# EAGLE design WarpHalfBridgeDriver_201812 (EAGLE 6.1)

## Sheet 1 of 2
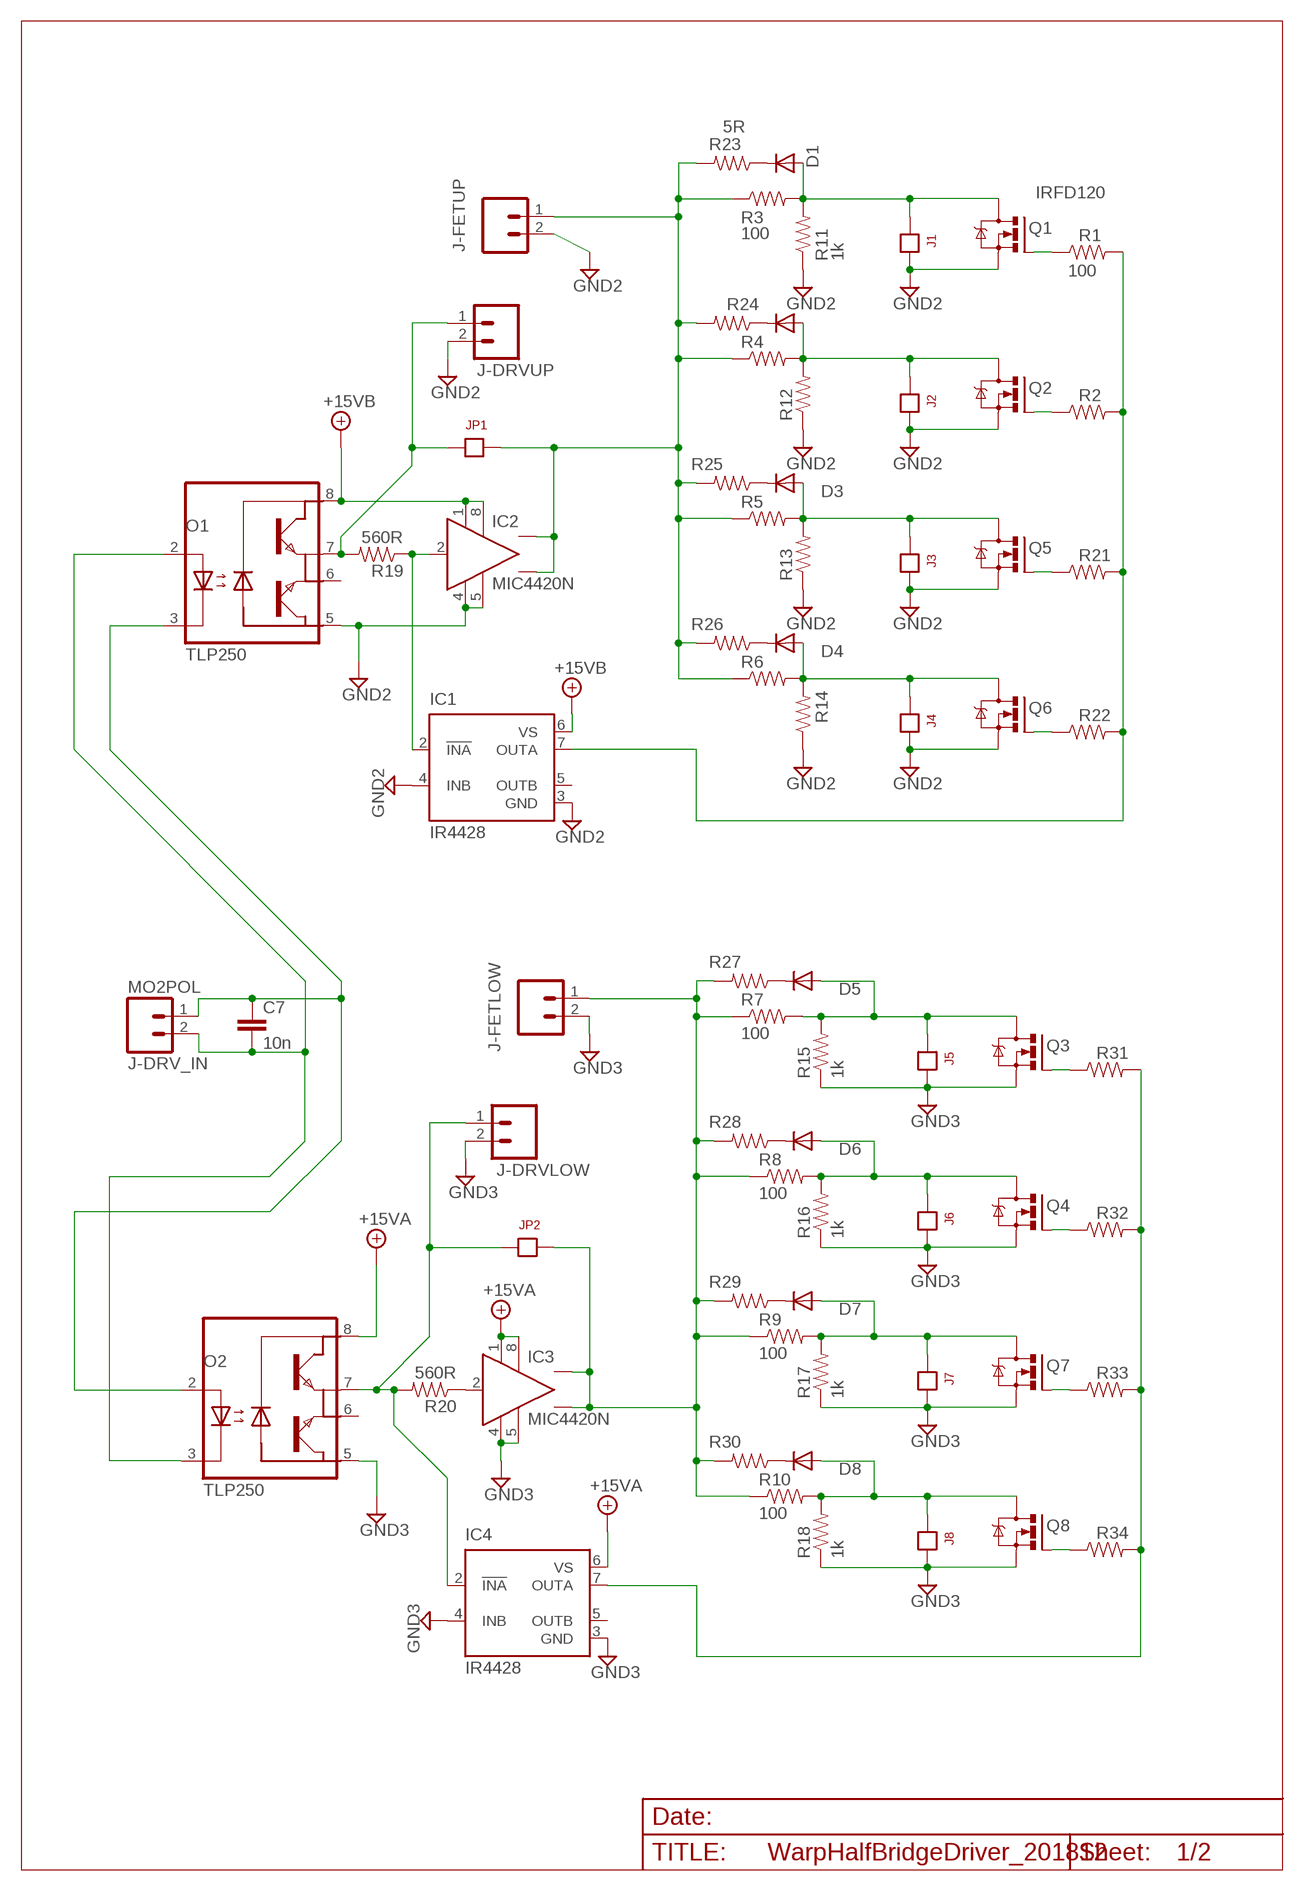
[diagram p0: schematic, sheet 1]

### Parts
C7  10n  BCAP  [BCAP]
D1  1N4004  [DO41-10]
D2  1N4004  [DO41-10]
D3  1N4004  [DO41-10]
D4  1N4004  [DO41-10]
D5  1N4004  [DO41-10]
D6  1N4004  [DO41-10]
D7  1N4004  [DO41-10]
D8  1N4004  [DO41-10]
IC1  IR4428  [DIL08]
IC2  MIC4420N  [DIL08]
IC3  MIC4420N  [DIL08]
IC4  IR4428  [DIL08]
J1  JP1  [JP1]
J2  JP1  [JP1]
J3  JP1  [JP1]
J4  JP1  [JP1]
J5  JP1  [JP1]
J6  JP1  [JP1]
J7  JP1  [JP1]
J8  JP1  [JP1]
J-DRV_IN  MO2POL  [MOLEX-1X2]
J-DRVLOW  MO2POL  [MOLEX-1X2]
J-DRVUP  MO2POL  [MOLEX-1X2]
J-FETLOW  MO2POL  [MOLEX-1X2]
J-FETUP  MO2POL  [MOLEX-1X2]
JP1  JP1  [JP1]
JP2  JP1  [JP1]
O1  TLP250  TLP250DIP8-L39  [DIL08-L39]
O2  TLP250  TLP250DIP8-L39  [DIL08-L39]
Q1  IRFD120  [DIL04]
Q2  IRFD120  [DIL04]
Q3  IRFD120  [DIL04]
Q4  IRFD120  [DIL04]
Q5  IRFD120  [DIL04]
Q6  IRFD120  [DIL04]
Q7  IRFD120  [DIL04]
Q8  IRFD120  [DIL04]
R1  100  RESISTORPTH-1/4W  [AXIAL-0.4]
R2  100  RESISTORPTH-1/4W  [AXIAL-0.4]
R3  100  RESISTORPTH-1/4W  [AXIAL-0.4]
R4  100  RESISTORPTH-1/4W  [AXIAL-0.4]
R5  100  RESISTORPTH-1/4W  [AXIAL-0.4]
R6  100  RESISTORPTH-1/4W  [AXIAL-0.4]
R7  100  RESISTORPTH-1/4W  [AXIAL-0.4]
R8  100  RESISTORPTH-1/4W  [AXIAL-0.4]
R9  100  RESISTORPTH-1/4W  [AXIAL-0.4]
R10  100  RESISTORPTH-1/4W  [AXIAL-0.4]
R11  1k  R4  [AXIAL-0.4]
R12  1k  R4  [AXIAL-0.4]
R13  1k  R4  [AXIAL-0.4]
R14  1k  R4  [AXIAL-0.4]
R15  1k  R4  [AXIAL-0.4]
R16  1k  R4  [AXIAL-0.4]
R17  1k  R4  [AXIAL-0.4]
R18  1k  R4  [AXIAL-0.4]
R19  560R  R4  [AXIAL-0.4]
R20  560R  R4  [AXIAL-0.4]
R21  100  RESISTORPTH-1/4W  [AXIAL-0.4]
R22  100  RESISTORPTH-1/4W  [AXIAL-0.4]
R23  5R  R4  [AXIAL-0.4]
R24  5R  R4  [AXIAL-0.4]
R25  5R  R4  [AXIAL-0.4]
R26  5R  R4  [AXIAL-0.4]
R27  5R  R4  [AXIAL-0.4]
R28  5R  R4  [AXIAL-0.4]
R29  5R  R4  [AXIAL-0.4]
R30  5R  R4  [AXIAL-0.4]
R31  100  RESISTORPTH-1/4W  [AXIAL-0.4]
R32  100  RESISTORPTH-1/4W  [AXIAL-0.4]
R33  100  RESISTORPTH-1/4W  [AXIAL-0.4]
R34  100  RESISTORPTH-1/4W  [AXIAL-0.4]

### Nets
+15VA: IC3.1(VS) IC3.8(VS1) IC4.6(VS) O2.8(VCC) ; also sheet 2
+15VB: IC1.6(VS) IC2.1(VS) IC2.8(VS1) O1.8(VCC) ; also sheet 2
GND2: IC1.3(GND) IC1.4(INB) IC2.4(GND) IC2.5(GND1) J1.2 J2.2 J3.2 J4.2 J-DRVUP.2 J-FETUP.2 O1.5(GND) Q1.4(S) Q2.4(S) Q5.4(S) Q6.4(S) R11.P$1 R12.P$1 R13.P$1 R14.P$1 ; also sheet 2
GND3: IC3.4(GND) IC3.5(GND1) IC4.3(GND) IC4.4(INB) J5.2 J6.2 J7.2 J8.2 J-DRVLOW.2 J-FETLOW.2 O2.5(GND) Q3.4(S) Q4.4(S) Q7.4(S) Q8.4(S) R15.P$1 R16.P$1 R17.P$1 R18.P$1 ; also sheet 2
N$1: C7.1 J-DRV_IN.1 O1.3(C) O2.2(A)
N$2: D2.A J2.1 Q2.1(D) R4.P$2 R12.P$2
N$3: D1.A J1.1 Q1.1(D) R3.P$2 R11.P$2
N$4: D1.C R23.P$1
N$5: IC1.2(!INA) IC2.2(IN) R19.P$1
N$7: Q1.3(G) R1.P$1
N$8: D6.A J6.1 Q4.1(D) R8.P$2 R16.P$2
N$9: D3.A J3.1 Q5.1(D) R5.P$2 R13.P$2
N$10: D4.A J4.1 Q6.1(D) R6.P$2 R14.P$2
N$11: IC4.2(!INA) J-DRVLOW.1 JP2.1 O2.7(VO2) R20.P$2
N$12: D5.A J5.1 Q3.1(D) R7.P$2 R15.P$2
N$13: D7.A J7.1 Q7.1(D) R9.P$2 R17.P$2
N$14: D8.A J8.1 Q8.1(D) R10.P$2 R18.P$2
N$15: J-DRVUP.1 JP1.1 O1.7(VO2) R19.P$2
N$16: IC3.2(IN) R20.P$1
N$17: Q2.3(G) R2.P$1
N$18: IC1.7(OUTA) R1.P$2 R2.P$2 R21.P$2 R22.P$2
N$19: Q5.3(G) R21.P$1
N$21: D2.C R24.P$1
N$22: Q6.3(G) R22.P$1
N$23: C7.2 J-DRV_IN.2 O1.2(A) O2.3(C)
N$24: D3.C R25.P$1
N$25: D4.C R26.P$1
N$27: IC2.6(OUT) IC2.7(OUT) J-FETUP.1 JP1.2 R3.P$1 R4.P$1 R5.P$1 R6.P$1 R23.P$2 R24.P$2 R25.P$2 R26.P$2
N$28: D5.C R27.P$1
N$30: IC3.6(OUT) IC3.7(OUT) J-FETLOW.1 JP2.2 R7.P$1 R8.P$1 R9.P$1 R10.P$1 R27.P$2 R28.P$2 R29.P$2 R30.P$2
N$31: D6.C R28.P$1
N$34: D7.C R29.P$1
N$37: D8.C R30.P$1
N$39: Q3.3(G) R31.P$1
N$41: Q4.3(G) R32.P$1
N$43: Q7.3(G) R33.P$1
N$45: Q8.3(G) R34.P$1
N$46: IC4.7(OUTA) R31.P$2 R32.P$2 R33.P$2 R34.P$2
Unconnected: IC1.5(OUTB) IC4.5(OUTB) O1.6(VO) O2.6(VO)

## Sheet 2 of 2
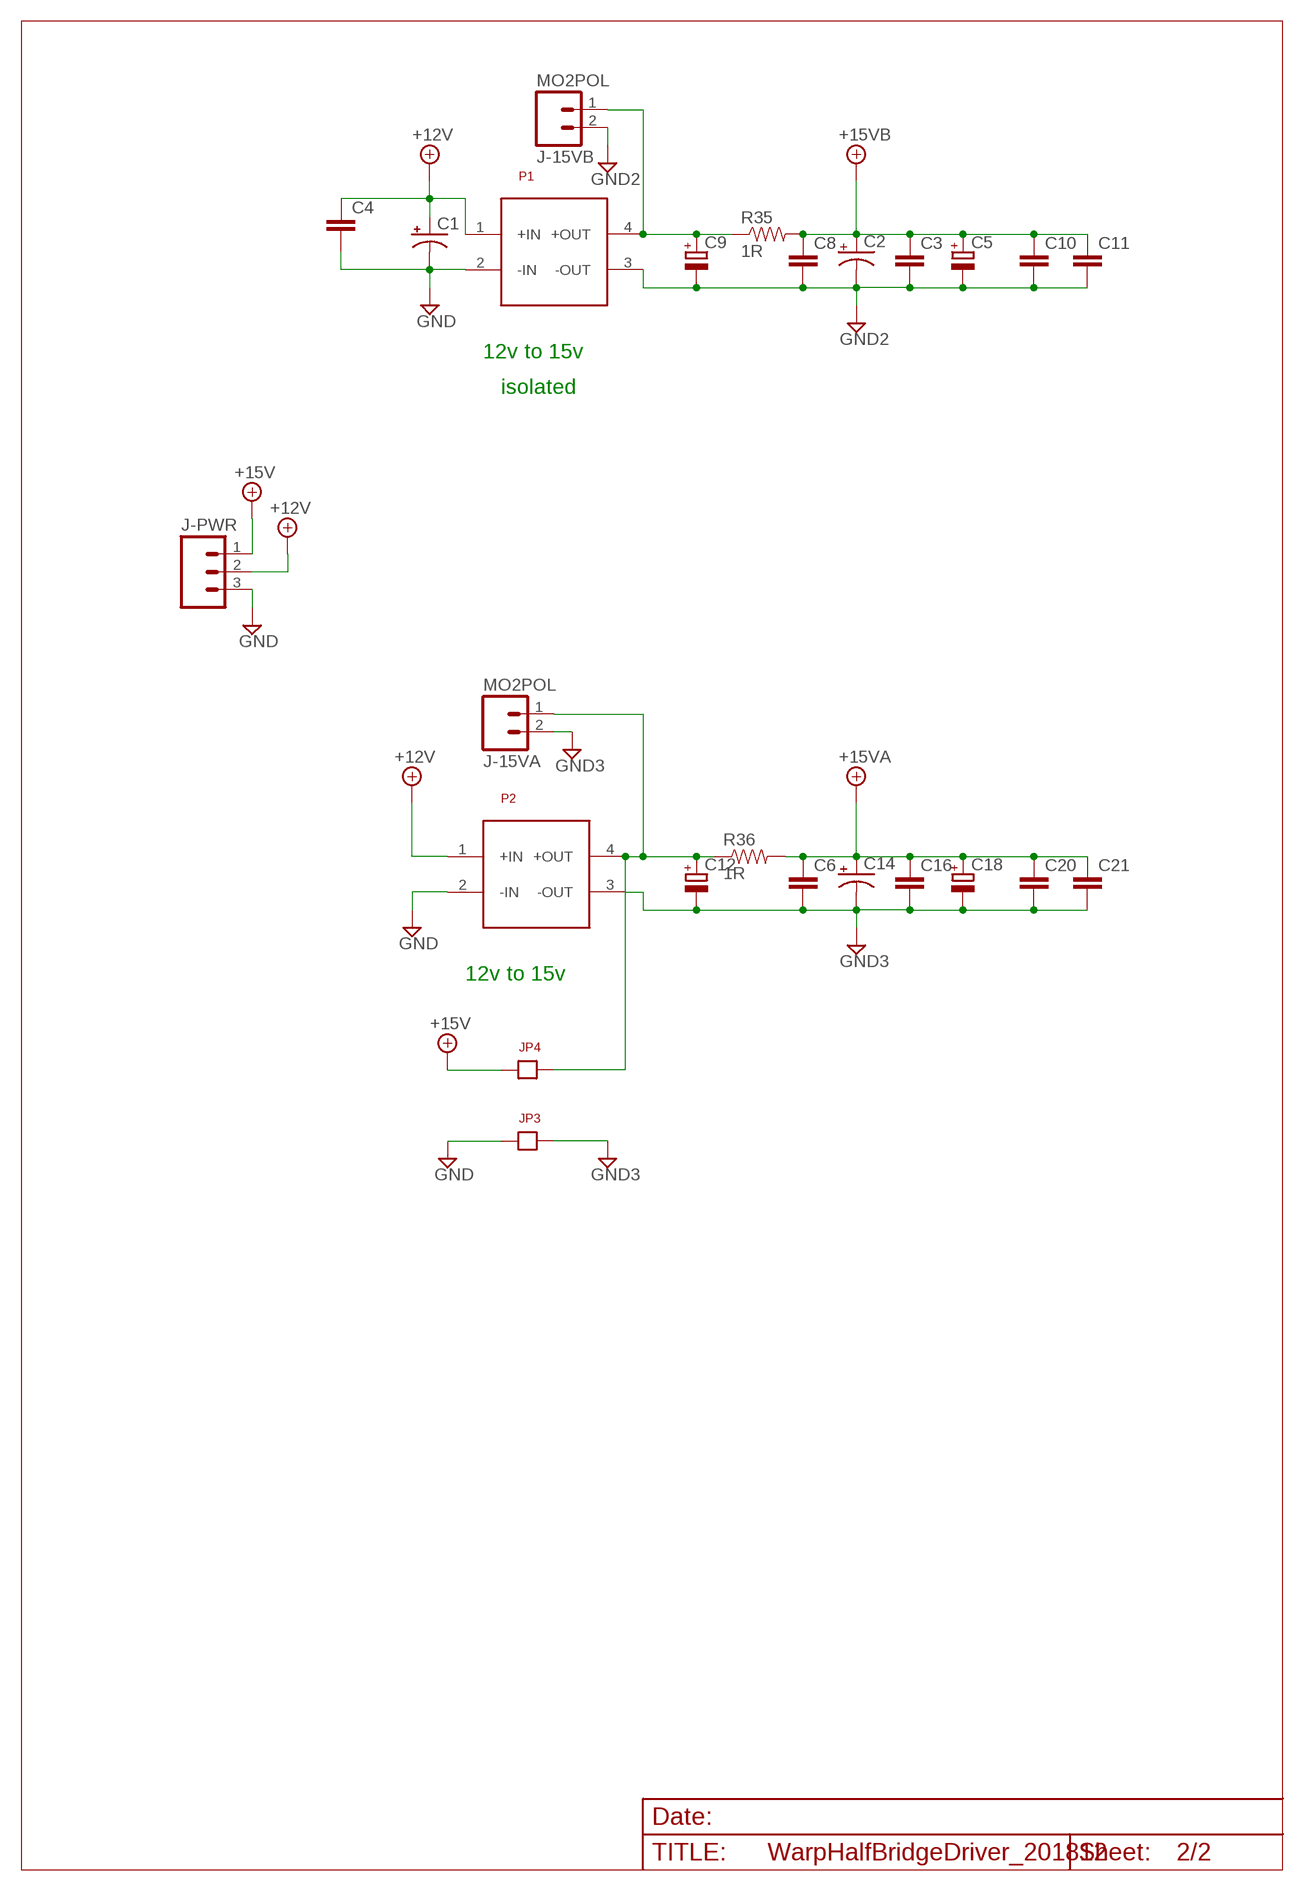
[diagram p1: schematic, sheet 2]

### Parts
C1  CAP_POLPTH1  [CPOL-RADIAL-100UF-25V]
C2  CAP_POLPTH1  [CPOL-RADIAL-100UF-25V]
C3  BCAP  [BCAP]
C4  BCAP  [BCAP]
C5  C-RB200100  [CPOL-RADIAL-10UF-25V]
C6  BCAP  [BCAP]
C8  BCAP  [BCAP]
C9  C-RB200100  [CPOL-RADIAL-10UF-25V]
C10  BCAP  [BCAP]
C11  BCAP  [BCAP]
C12  C-RB200100  [CPOL-RADIAL-10UF-25V]
C14  CAP_POLPTH1  [CPOL-RADIAL-100UF-25V]
C16  BCAP  [BCAP]
C18  C-RB200100  [CPOL-RADIAL-10UF-25V]
C20  BCAP  [BCAP]
C21  BCAP  [BCAP]
J-15VA  MO2POL  [MOLEX-1X2]
J-15VB  MO2POL  [MOLEX-1X2]
J-PWR  MO3POL  [MOLEX-3]
JP3  JP1  [JP1]
JP4  JP1  [JP1]
P1  VFSD-S12-S12  VFSD-S5-S12  [VFSD2]
P2  VFSD-S12-S12  VFSD-S5-S12  [VFSD2]
R35  1R  R4  [AXIAL-0.4]
R36  1R  R4  [AXIAL-0.4]

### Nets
+12V: C1.1(+) C4.1 J-PWR.2 P1.1(+IN) P2.1(+IN)
+15V: J-PWR.1 JP4.1
+15VA: C6.1 C14.1(+) C16.1 C18.1(+) C20.1 C21.1 R36.P$2 ; also sheet 1
+15VB: C2.1(+) C3.1 C5.1(+) C8.1 C10.1 C11.1 R35.P$2 ; also sheet 1
GND: C1.2(-) C4.2 J-PWR.3 JP3.1 P1.2(-IN) P2.2(-IN)
GND2: C2.2(-) C3.2 C5.2(-) C8.2 C9.2(-) C10.2 C11.2 J-15VB.2 P1.3(-OUT) ; also sheet 1
GND3: C6.2 C12.2(-) C14.2(-) C16.2 C18.2(-) C20.2 C21.2 J-15VA.2 JP3.2 P2.3(-OUT) ; also sheet 1
N$6: C12.1(+) J-15VA.1 JP4.2 P2.4(+OUT) R36.P$1
N$20: C9.1(+) J-15VB.1 P1.4(+OUT) R35.P$1

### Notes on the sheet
- 12v to 15v
- isolated
- 12v to 15v

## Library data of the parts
C1 C2 C14 = SparkFun-Passives:CAP_POL: Capacitor Polarized
C3 C4 C6 C8 C10 C11 C16 C20 C21 = Andrew Misc:BCAP
C5 C9 C12 C18 = Andrew:C-RB200100
C7 = Andrew junk:BCAP
D1-D8 = diode:1N4004: DIODE
IC1 IC4 = ir:IR4428: DUAL LOW SIDE DRIVER Source: ID4426.pdf; MF: INTERNATIONAL RECTIFIER(IR); MPN: IR4428PBF; OC_FARNELL: 1023268; OC_NEWARK: 19K8464
IC2 IC3 = Andrew IC:MIC4420: 6A-Peak Low-Side MOSFET Driver Bipolar/CMOS/DMOS Process http://www.micrel.com/_PDF/mic4420.pdf
J1-J8 JP1 JP2 = Andrew Connectors:JP1
J-15VA J-15VB J-DRV_IN J-DRVLOW J-DRVUP J-FETLOW J-FETUP = Andrew_Connectors:MO2POL
J-PWR = Andrew_Connectors:MO3POL
JP3 JP4 = Andrew_Connectors:JP1
O1 O2 = Andrew IC:TLP250: HEWLETT PACKARD OPTO COUPLER
P1 P2 = Andrew ISOPWR:VFSD-S5-S12
Q1-Q8 = Andrew Transistor:IRFD120
R1-R10 R21 R22 R31-R34 = SparkFun-Passives:RESISTOR: Resistor
R11-R20 R23-R30 R35 R36 = Andrew Misc:R4

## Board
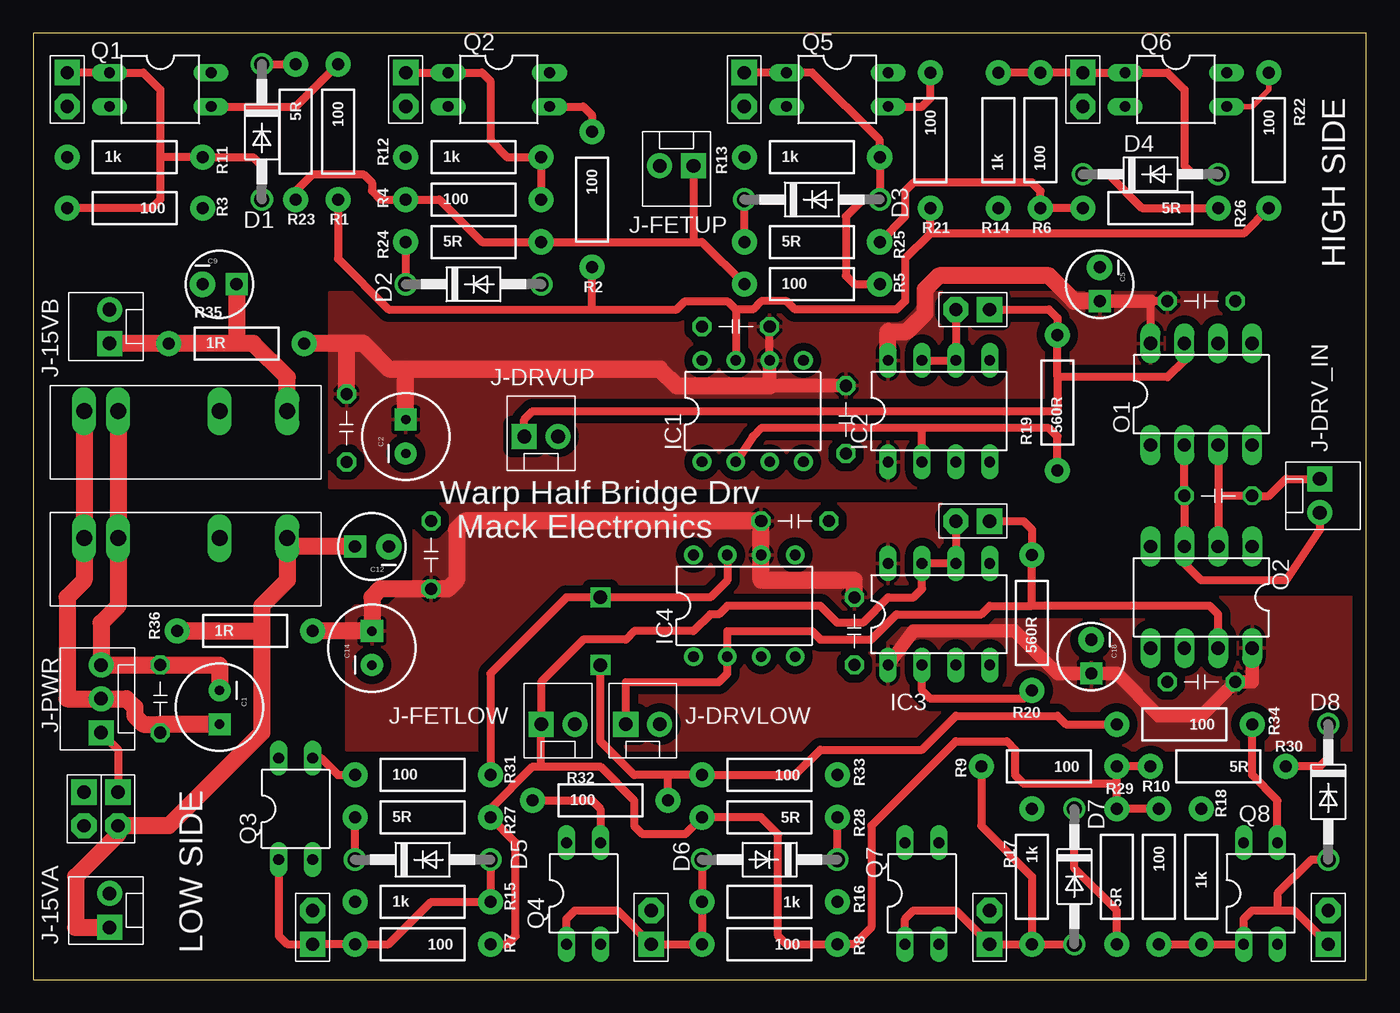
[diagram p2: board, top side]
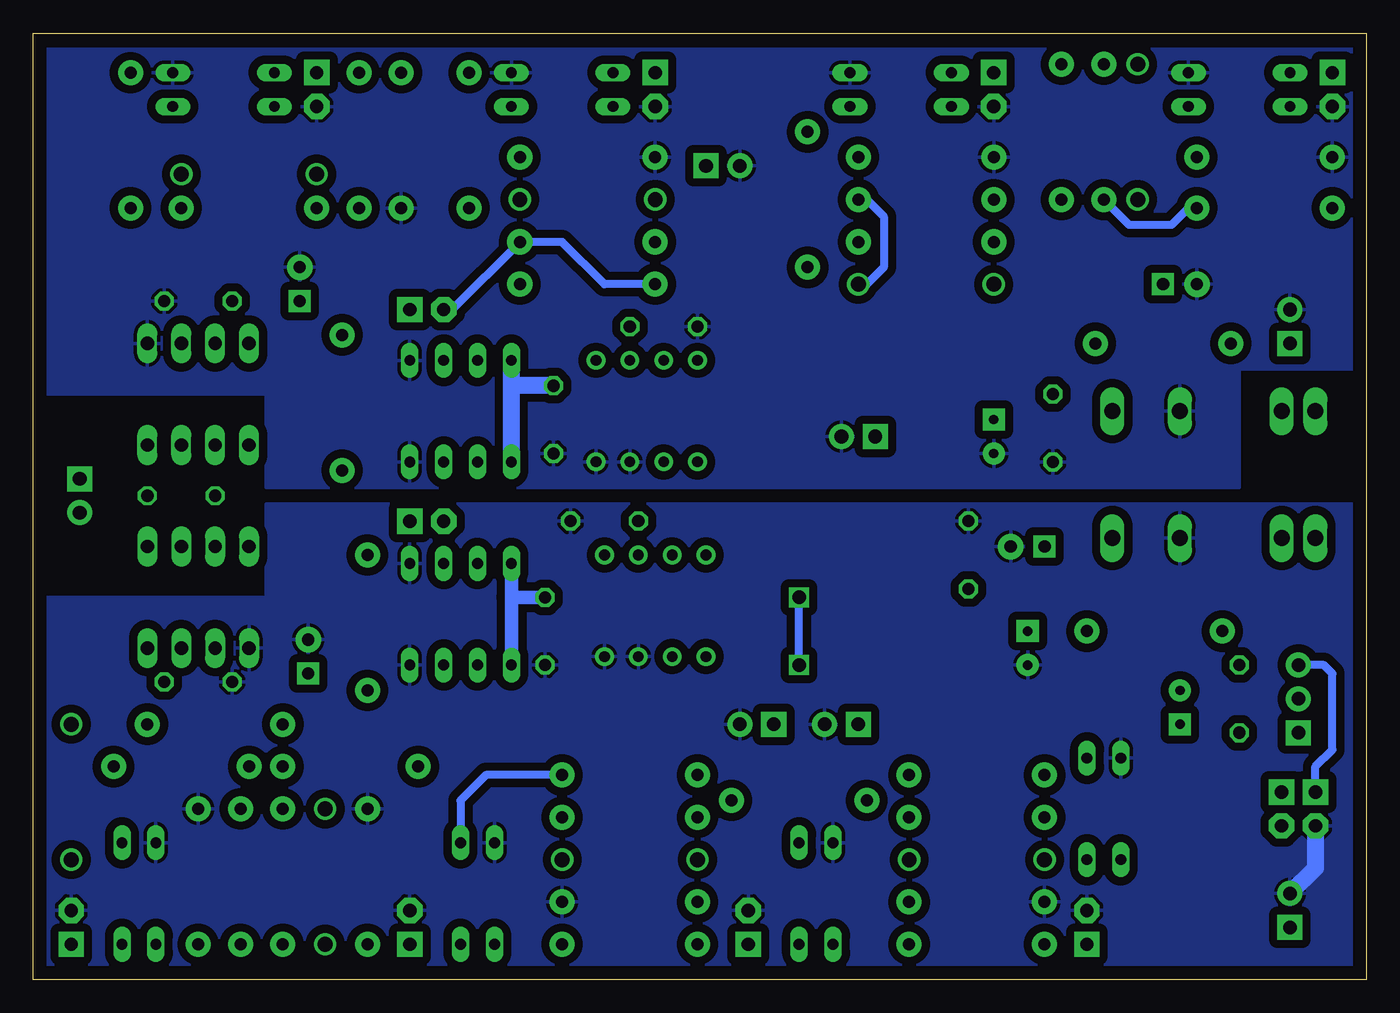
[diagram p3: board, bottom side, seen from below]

Size 100 x 71 mm. Coordinates in mm from the lower left corner, seen from the top.
Outline: 0,0 100,0 100,71 0,71 0,0
Copper layers (1*16): Top 0.035mm / dielectric 1.5mm / Bottom 0.035mm
Design rules: minimum track width 10mil, minimum drill 24mil, track to track 10mil, track to pad 10mil, pad to pad 10mil, via to via 10mil, smd to smd 8mil, copper to edge 40mil, drill to drill 8mil, minimum pad ring 10mil, minimum via ring 8mil, stop-mask expansion 4mil, vias tented up to drill 0mil, thermal gap 10mil

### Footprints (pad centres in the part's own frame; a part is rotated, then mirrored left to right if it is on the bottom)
CPOL-RADIAL-100UF-25V = drill 0.7 pad 1.651 square: 1 1.27,0 | drill 0.7 pad 1.651: 2 -1.27,0
BCAP = drill 0.914 octagon: 1 -2.54,0; 2 2.54,0
CPOL-RADIAL-10UF-25V = drill 0.914 pad 1.651 square: 1 1.27,0 | drill 0.914 pad 1.905: 2 -1.27,0
DO41-10 = drill 1.118: A 5.08,0; C -5.08,0
DIL08 = drill 0.8 pad 1.4: 1 -3.81,-3.81; 2 -1.27,-3.81; 3 1.27,-3.81; 4 3.81,-3.81; 5 3.81,3.81; 6 1.27,3.81; 7 -1.27,3.81; 8 -3.81,3.81
DIL08' = drill 0.813 long: 1 -3.81,-3.81; 2 -1.27,-3.81; 3 1.27,-3.81; 4 3.81,-3.81; 5 3.81,3.81; 6 1.27,3.81; 7 -1.27,3.81; 8 -3.81,3.81
JP1 = drill 1 pad 1.905 square: 1 -1.27,0 | drill 1 pad 1.905 octagon: 2 1.27,0
MOLEX-1X2 = drill 1.016 pad 1.88 square: 1 0,0 | drill 1.016 pad 1.88: 2 2.54,0
MOLEX-3 = drill 1.016 pad 1.88 square: 1 -2.54,0 | drill 1.016 pad 1.88: 2 0,0; 3 2.54,0
DIL08-L39 = drill 1 long: 1 -3.81,-3.81; 2 -1.27,-3.81; 3 1.27,-3.81; 4 3.81,-3.81; 5 3.81,3.81; 6 1.27,3.81; 7 -1.27,3.81; 8 -3.81,3.81
VFSD2 = drill 1.2 long: 1 -3.81,0; 2 -1.27,0; 3 6.35,0; 4 11.43,0
DIL04 = drill 0.813 long: 1 -1.27,-3.81; 2 1.27,-3.81; 3 1.27,3.81; 4 -1.27,3.81
AXIAL-0.4 = drill 0.9 pad 1.88: P$1 -5.08,0; P$2 5.08,0

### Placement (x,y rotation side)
C1  13.97,20.42 270 top
C2  27.94,40.74 90 top
C3  23.5,41.38 270 top
C4  9.53,21.06 90 top
C5  80.01,52.17 270 top
C6  57.15,34.4 0 top
C7  88.9,36.3 180 top
C8  60.96,42.02 270 top
C9  13.97,52.17 0 top
C10  52.7,49 180 top
C11  87.63,50.91 0 top
C12  25.4,32.49 180 top
C14  25.4,24.87 90 top
C16  61.59,26.14 270 top
C18  79.38,24.23 270 top
C20  87.63,22.33 180 top
C21  29.84,31.85 90 top
D1  17.14,63.61 270 top
D2  33.02,52.17 0 top
D3  58.42,58.53 0 top
D4  83.82,60.43 0 top
D5  29.21,9 0 top
D6  55.24,9 180 top
D7  78.11,7.73 270 top
D8  97.16,14.07 270 top
IC1  53.98,42.65 0 top
IC2  MIC4420N  [DIL08']  67.94,42.65 0 top
IC3  MIC4420N  [DIL08']  67.94,27.41 0 top
IC4  53.34,28.05 0 top
J1  2.54,66.78 270 top
J2  27.94,66.78 270 top
J3  53.34,66.78 270 top
J4  78.74,66.78 270 top
J5  20.95,3.91 90 top
J6  46.35,3.91 90 top
J7  71.75,3.91 90 top
J8  97.16,3.91 90 top
J-15VA  5.71,3.91 90 top
J-15VB  5.71,47.73 90 top
J-DRV_IN  96.52,37.57 270 top
J-DRVLOW  44.45,19.16 0 top
J-DRVUP  36.83,40.74 0 top
J-FETLOW  38.1,19.16 0 top
J-FETUP  49.53,61.06 180 top
J-PWR  5.08,21.06 90 top
JP1  70.48,50.27 180 top
JP2  70.48,34.4 180 top
JP3  3.81,12.8 270 top
JP4  6.35,12.8 270 top
O1  87.63,43.92 0 top
O2  87.63,28.68 180 top
P1  7.62,42.65 0 top
P2  7.62,33.12 0 top
Q1  9.53,66.78 270 top
Q2  34.92,66.78 270 top
Q3  19.68,12.8 0 top
Q4  41.27,6.45 0 top
Q5  60.33,66.78 270 top
Q6  85.72,66.78 270 top
Q7  66.67,6.45 0 top
Q8  92.08,6.45 0 top
R1  22.86,63.61 270 top
R2  41.91,58.53 270 top
R3  7.62,57.89 180 top
R4  33.02,58.53 0 top
R5  58.42,52.17 0 top
R6  75.56,62.97 90 top
R7  29.21,2.64 180 top
R8  55.24,2.64 180 top
R9  76.2,15.98 180 top
R10  84.45,7.73 270 top
R11  7.62,61.7 0 top
R12  33.02,61.7 0 top
R13  58.42,61.7 0 top
R14  72.39,62.97 90 top
R15  29.21,5.82 0 top
R16  55.24,5.82 180 top
R17  74.93,7.73 270 top
R18  87.63,7.73 270 top
R19  76.83,43.28 90 top
R20  74.93,26.77 90 top
R21  67.31,62.97 270 top
R22  92.71,62.97 270 top
R23  19.68,63.61 270 top
R24  33.02,55.35 0 top
R25  58.42,55.35 0 top
R26  83.82,57.89 180 top
R27  29.21,12.17 0 top
R28  55.24,12.17 180 top
R29  81.28,7.73 90 top
R30  88.9,15.98 180 top
R31  29.21,15.34 0 top
R32  42.55,13.44 0 top
R33  55.24,15.34 180 top
R34  86.36,19.16 180 top
R35  15.24,47.73 0 top
R36  15.88,26.14 0 top

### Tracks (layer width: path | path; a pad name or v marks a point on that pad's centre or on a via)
+12V
  Top 1.27: P1.1 P2.1 3.81,29.95 2.54,28.68 2.54,21.06 J-PWR.2 6.99,21.06 7.62,20.42 7.62,19.79 8.26,19.16 9.53,19.16 | C1.1 9.53,19.16 | 9.53,19.16 C4.1
+15V
  Top 0.61: J-PWR.1 6.35,17.25 JP4.1
+15VA
  Top 1.016: O2.8 91.44,22.33 C20.1 87.63,19.79 84.45,19.79 81.28,22.97 C18.1 76.83,22.97 73.66,26.14 66.04,26.14 IC3.1
  Top 1.27: C16.1 61.59,29.95 54.61,29.95 IC4.6 C6.1 32.38,34.4 31.75,33.76 31.75,29.95 31.11,29.31 C21.1 26.04,29.31 25.4,28.68 C14.1 R36.P$2
  Bottom 1.016: IC3.8 64.14,28.68 | 64.14,28.68 IC3.1 | C16.1 64.14,28.68
  pour Top (isolate 0.61): 28.57,35.66 28.57,29.95 26.67,28.05 24.13,28.05 23.5,27.41 23.5,17.25 99.06,17.25 99.06,28.68 81.92,28.68 81.92,35.66
+15VB
  Top 0.61: C11.1 83.82,50.91 O1.8 | IC1.6 C10.1
  Top 1.016: 83.82,50.91 C5.1 | IC1.6 55.24,44.55 C8.1
  Top 1.27: 27.94,45.83 26.67,45.83 24.77,47.73 23.5,47.73 | 27.94,45.83 46.99,45.83 48.26,44.55 55.24,44.55 | 23.5,47.73 R35.P$2 | C3.1 23.5,47.73 | C2.1 27.94,45.83 | C5.1 78.11,50.91 76.2,52.81 67.94,52.81 66.93,51.79 66.93,50.02 65.53,48.62 64.14,48.62 IC2.8
  Bottom 1.27: IC2.1 64.14,44.55 | 64.14,44.55 IC2.8 | C8.1 64.14,44.55
  pour Top (isolate 0.61): 22.23,36.94 22.23,51.54 99.06,51.54 99.06,43.92 82.55,43.92 82.55,36.94
GND
  Top 1.27: P1.2 P2.2 6.35,28.05 5.08,26.77 J-PWR.3 C4.2 13.97,23.6 C1.2
  Bottom 0.61: JP3.1 3.81,15.98 2.54,17.25 2.54,22.97 3.17,23.6 J-PWR.3
GND2
  pour Bottom (isolate 0.61): 0.64,69.95 99.69,69.95 99.69,69.32 99.69,43.92 82.55,43.92 82.55,36.94 9.53,36.94 9.53,38.2 9.53,45.83 0.64,45.83
GND3
  Bottom 1.27: JP3.2 3.81,8.36 J-15VA.2
  pour Bottom (isolate 0.61): 0.64,35.66 82.55,35.66 82.55,28.68 99.69,28.68 99.69,0.74 0.64,0.74
N$1
  Top 0.61: O1.3 88.9,36.3 | 88.9,36.3 O2.2 | 88.9,36.3 C7.1 92.71,36.3 93.98,37.57 J-DRV_IN.1
N$2
  Top 0.61: J2.1 Q2.1 33.66,68.05 34.29,67.42 34.29,62.97 35.56,61.7 R12.P$2 R4.P$2
  Bottom 0.61: R4.P$2 37.47,58.53 36.2,57.25 36.2,53.44 37.47,52.17 D2.A
N$3
  Top 0.61: J1.1 Q1.1 8.26,68.05 9.53,66.78 9.53,61.7 | 9.53,61.7 9.53,58.53 8.89,57.89 R3.P$2 | 9.53,61.7 R11.P$2 16.51,61.7 17.14,61.06 D1.A
N$4
  Top 0.61: D1.C R23.P$1
N$5
  Top 0.61: R19.P$1 76.83,40.74 76.2,41.38 66.67,41.38 | 66.67,41.38 54.61,41.38 53.98,40.74 IC1.2 | IC2.2 66.67,41.38
N$6
  Top 0.61: 17.14,28.05 17.14,26.77 16.51,26.14
  Top 1.27: P2.4 19.05,32.49 | 13.97,26.14 R36.P$1 16.51,26.14 | J-15VA.1 3.17,3.91 3.17,7.73 6.35,10.9 JP4.2 10.16,11.54 17.14,18.52 17.14,28.05 19.05,29.95 19.05,32.49 | C12.1 19.05,32.49
N$7
  Top 0.61: Q1.3 19.68,65.51 R1.P$1
N$8
  Top 0.61: Q4.1 40.01,4.55 40.64,5.18 43.81,5.18 J6.1 R8.P$2 R16.P$2 D6.A
N$9
  Top 0.61: J3.1 Q5.1 58.42,68.05 63.5,62.97 R13.P$2 D3.A 62.23,58.53 60.96,57.25 60.96,52.81 61.59,52.17 R5.P$2
N$10
  Top 0.61: Q6.1 J4.1 R6.P$2 R14.P$2 | 82.55,68.05 Q6.1 | Q6.1 85.09,68.05 86.36,66.78 86.36,61.06 87,60.43 D4.A
N$11
  Top 0.61: O2.7 88.9,27.41 88.27,28.05 74.93,28.05 | 74.93,28.05 R20.P$2 74.93,33.76 74.3,34.4 JP2.1 | J-DRVLOW.1 44.45,22.33 51.44,22.33 52.07,22.97 IC4.2 52.07,26.14 58.42,26.14 59.05,25.51 62.87,25.51 64.77,27.41 71.12,27.41 71.75,28.05 74.93,28.05
N$12
  Top 0.61: Q3.1 18.41,3.28 19.05,2.64 J5.1 R7.P$2 26.67,2.64 29.84,5.82 R15.P$2 D5.A
N$13
  Top 0.61: Q7.1 65.41,4.55 66.04,5.18 69.22,5.18 J7.1 R17.P$2 | R17.P$2 D7.A | R9.P$2 71.12,11.54 74.93,7.73 R17.P$2
N$14
  Top 0.61: R10.P$2 R18.P$2 Q8.1 90.81,4.55 91.44,5.18 93.34,5.18 | 93.34,5.18 94.61,5.18 J8.1 | D8.A 95.89,9 93.34,6.45 93.34,5.18
N$15
  Top 0.61: O1.7 86.36,46.46 85.09,45.19 76.83,45.19 | 76.83,45.19 R19.P$2 76.83,49.64 76.2,50.27 JP1.1 | J-DRVUP.1 36.83,42.02 37.47,42.65 76.83,42.65 76.83,45.19
N$16
  Top 0.61: R20.P$1 74.3,21.06 67.31,21.06 66.67,21.7 IC3.2
N$17
  Top 0.61: Q2.3 41.27,65.51 41.91,64.88 R2.P$1
N$18
  Top 0.61: R22.P$2 90.81,55.98 67.31,55.98 | 67.31,55.98 R21.P$2 | R1.P$2 22.86,54.08 26.67,50.27 41.91,50.27 | 41.91,50.27 R2.P$2 | 41.91,50.27 48.26,50.27 48.9,50.91 52.07,50.91 52.7,50.27 | 52.7,50.27 IC1.7 | 52.7,50.27 53.98,50.27 54.61,50.91 56.52,50.91 57.15,50.27 64.77,50.27 65.41,50.91 65.41,54.08 67.31,55.98
N$19
  Top 0.61: Q5.3 66.67,65.51 67.31,66.14 R21.P$1
N$20
  Top 1.27: P1.4 19.05,45.19 16.51,47.73 15.24,47.73 | 15.24,47.73 R35.P$1 J-15VB.1 | C9.1 15.24,47.73
N$21
  Top 0.61: R24.P$1 D2.C
N$22
  Top 0.406: R22.P$1 92.71,66.78 91.44,65.51 Q6.3
N$23
  Top 0.61: O1.2 C7.2 O2.3 86.36,31.22 87.63,29.95 93.98,29.95 96.52,33.76 J-DRV_IN.2
N$24
  Top 0.61: R25.P$1 D3.C
N$25
  Top 0.61: D4.C 80.64,60.43 83.19,57.89 R26.P$1
N$27
  Top 0.61: 49.53,55.35 R24.P$2 33.66,55.35 30.48,58.53 R4.P$1 26.04,58.53 25.4,59.16 25.4,59.8 24.77,60.43 20.95,60.43 19.68,59.16 R23.P$2 | 49.53,55.35 50.16,55.35 R5.P$1 | R26.P$2 R6.P$1 75.56,59.16 74.93,59.8 66.04,59.8 65.41,59.16 65.41,57.25 R25.P$2 | JP1.2 IC2.6 IC2.7 | J-FETUP.1 49.53,55.35
  Bottom 0.61: R3.P$1 13.34,57.89 14.61,56.62 17.78,56.62 R23.P$2 | R5.P$1 57.15,52.17 60.33,55.35 R25.P$2 68.58,50.27 JP1.2
N$28
  Top 0.61: D5.C R27.P$1
N$30
  Top 0.61: R30.P$2 R9.P$1 81.28,14.71 | R10.P$1 R29.P$2 81.28,14.71 | R7.P$1 35.56,2.64 36.2,3.28 36.2,10.27 R27.P$2 34.29,12.8 37.47,15.98 38.1,15.98 | 38.1,15.98 J-FETLOW.1 38.1,22.33 41.27,25.51 44.45,25.51 45.09,26.14 49.53,26.14 50.8,27.41 51.44,27.41 52.07,28.05 59.05,28.05 60.33,26.77 62.23,26.77 64.14,28.68 66.04,28.68 66.67,29.31 IC3.7 IC3.6 JP2.2 | 81.28,14.71 74.3,14.71 73.66,15.34 73.66,17.25 73.03,17.88 69.22,17.88 62.87,11.54 62.87,3.91 61.59,2.64 R8.P$1 56.52,2.64 55.88,3.28 55.88,10.9 54.61,12.17 R28.P$2 48.9,10.9 45.72,10.9 45.09,11.54 45.09,13.44 42.55,15.98 38.1,15.98
N$31
  Top 0.61: D6.C R28.P$1
N$34
  Top 0.61: R29.P$1 81.28,5.18 78.11,8.36 D7.C
N$37
  Top 0.61: D8.C 97.16,16.61 96.52,15.98 R30.P$1
N$39
  Top 0.61: Q3.3 21.59,16.61 22.86,15.34 R31.P$1
N$41
  Top 0.61: R32.P$1 41.91,13.44 42.55,12.8 Q4.3
N$43
  Bottom 0.61: R33.P$1 66.04,15.34 67.94,13.44 Q7.3
N$45
  Top 0.61: Q8.3 93.34,13.44 91.44,15.34 R34.P$1
N$46  (via drill 1)
  Top 0.61: 47.62,15.34 R33.P$2 57.15,15.34 59.05,17.25 66.67,17.25 69.22,19.79 76.83,19.79 77.47,19.16 R34.P$2 | IC4.7 52.07,29.95 50.8,28.68 v42.55,28.68 40.01,28.68 34.29,22.97 R31.P$2 | R32.P$2 47.62,15.34 | 47.62,15.34 45.09,15.34 42.55,17.88 v42.55,23.6
  Bottom 0.61: v42.55,23.6 v42.55,28.68

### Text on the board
tPlace: HIGH SIDE | Warp Half Bridge Drv | Mack Electronics | LOW SIDE

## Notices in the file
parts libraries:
SparkFun-Passives: Licensing: CC v3.0 Share-Alike You are welcome to use this library for commercial purposes.
